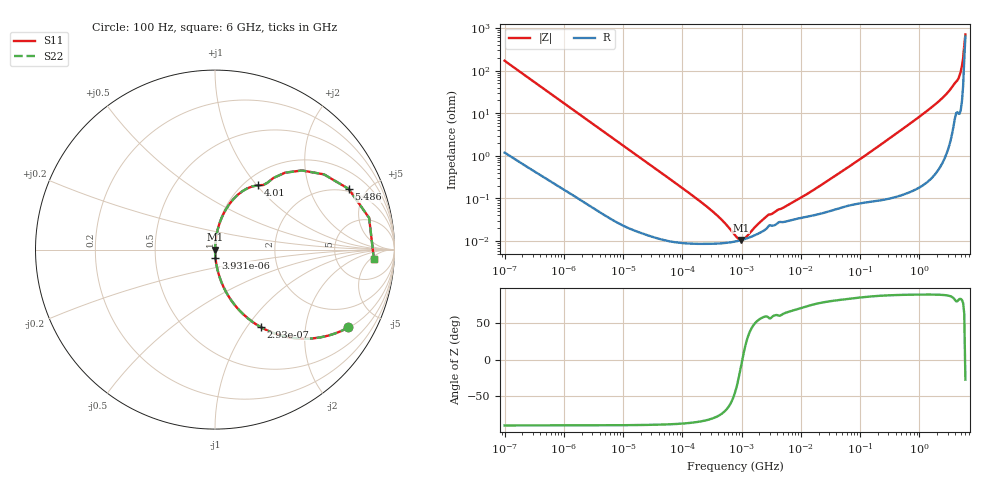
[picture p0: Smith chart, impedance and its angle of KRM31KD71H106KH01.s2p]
!Murata Part Number: KRM31KD71H106KH01
!These Parameters are Measured in Series Mode Connection
!Data Generated on Jan 08, 2026
!  o--ll--o
!Port1  Port2
!  o------o
!Operation Temp=25[degC], DC Bias Voltage=0[V]
!Freq. Start=100[Hz] Stop=6[GHz] 401[Steps]
# Hz S RI R 50
!Freq.(Hz) S11(Real) S11(Imag) S21(Real) S21(Imag) S12(Real) S12(Imag) S22(Real) S22(Imag)
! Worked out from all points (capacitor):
!   401 points, 100 Hz to 6 GHz, reference 50 ohm
!   read as one part in series: C = 9.3 uF near 109 Hz
!   lowest |Z| = 10.7 mohm at 969 kHz (marker M1)
!   series resonance near 1.029 MHz, so ESL is about 2.6 nH
!   S11 on the Smith chart (normalised r, x): 100 Hz: 1.02, -3.42; 293 Hz: 1.01, -1.17; 3.931 kHz: 1.00, -0.09; 4.01 GHz: 1.16, +1.02; 5.486 GHz: 1.84, +3.76; 6 GHz: 14, -6
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100  0.7432 -0.4334  0.2568 0.4334  0.2568 0.4334  0.7432 -0.4334
171  0.5003 -0.4963  0.4997 0.4963  0.4997 0.4963  0.5003 -0.4963
293  0.2574 -0.4333  0.7426 0.4333  0.7426 0.4333  0.2574 -0.4333
627  0.0722 -0.2544  0.9278 0.2544  0.9278 0.2544  0.0722 -0.2544
2008  0.00827 -0.0856  0.9917 0.0856  0.9917 0.0856  0.00827 -0.0856
3931  0.00245 -0.0442  0.9976 0.0442  0.9976 0.0442  0.00245 -0.0442
40335  0.000132 -0.00437  0.9999 0.00437  0.9999 0.00437  0.000132 -0.00437
302498  8.66e-05 -0.000533  0.9999 0.000533  0.9999 0.000533  8.66e-05 -0.000533
774597  9.76e-05 -9.68e-05  0.9999 9.68e-05  0.9999 9.68e-05  9.76e-05 -9.68e-05
968953  0.000105 -1.99e-05  0.9999 1.99e-05  0.9999 1.99e-05  0.000105 -1.99e-05
1159002  0.000113 3.94e-05  0.9999 -3.94e-05  0.9999 -3.94e-05  0.000113 3.94e-05
2713602  0.000205 0.000337  0.9998 -0.000337  0.9998 -0.000337  0.000205 0.000337
1.555665e7  0.000398 0.00146  0.9996 -0.00146  0.9996 -0.00146  0.000398 0.00146
3.124326e8  0.00164 0.0255  0.9984 -0.0255  0.9984 -0.0255  0.00164 0.0255
1.000774e9  0.00856 0.0819  0.9914 -0.0819  0.9914 -0.0819  0.00856 0.0819
2.142435e9  0.0398 0.1832  0.9602 -0.1832  0.9602 -0.1832  0.0398 0.1832
3.065283e9  0.1002 0.2783  0.8998 -0.2783  0.8998 -0.2783  0.1002 0.2783
4.009986e9  0.2415 0.3583  0.7585 -0.3583  0.7585 -0.3583  0.2415 0.3583
4.586474e9  0.3255 0.3992  0.6745 -0.3992  0.6745 -0.3992  0.3255 0.3992
5.016141e9  0.4847 0.441  0.5153 -0.441  0.5153 -0.441  0.4847 0.441
5.486059e9  0.7445 0.3384  0.2555 -0.3384  0.2555 -0.3384  0.7445 0.3384
6e9  0.8851 -0.0508  0.1149 0.0508  0.1149 0.0508  0.8851 -0.0508
